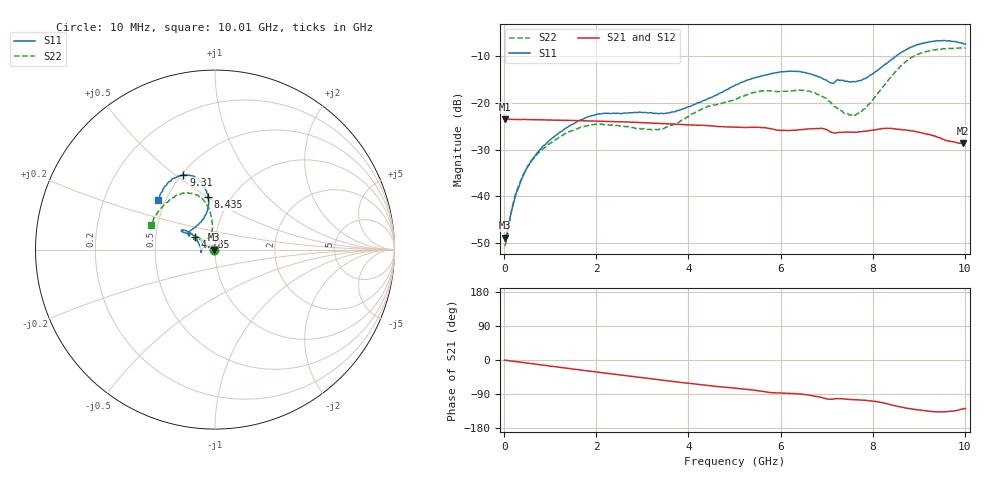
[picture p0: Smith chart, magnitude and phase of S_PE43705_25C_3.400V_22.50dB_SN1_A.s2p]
! Device ID: PE43705
! Serial: 1
! Insertion: A
! Impedance: 50 ohm
! Temp: 25C
! VDD: 3.400V
! Attenuation Step: 22.50dB
#  Hz  S  RI  R  50
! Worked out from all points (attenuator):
!   401 points, 10 MHz to 10.01 GHz, reference 50 ohm
!   highest |S21| = -23.53 dB at 10 MHz (marker M1); lowest = -28.7 dB at 9.96 GHz (marker M2)
!   lowest |S11| = -48.8 dB at 10 MHz (marker M3), VSWR 1.01, Z = 49.6 + j0.0396 ohm
!   |S11| at or under -10 dB: start of sweep to 8.518 GHz
!   |S22| runs from -50.6 to -8.3 dB; largest |S21 - S12| = 0.00078
!   S11 on the Smith chart (normalised r, x): 10 MHz: 0.99, +0.00; 4.785 GHz: 0.79, +0.12; 8.435 GHz: 0.79, +0.50; 9.31 GHz: 0.51, +0.53; 10.01 GHz: 0.45, +0.31
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1e7  -0.0036 0.000399  0.0666 -0.000213  0.0666 -0.000231  -0.00291 0.000506
6e7  -0.00344 0.00218  0.0664 -0.00125  0.0664 -0.00123  -0.00248 0.00251
2.6e8  -0.00513 0.00943  0.066 -0.00508  0.066 -0.00502  -0.00371 0.0104
5.35e8  -0.0124 0.0178  0.0652 -0.0102  0.0652 -0.0101  -0.00968 0.0192
1.01e9  -0.0346 0.0214  0.0626 -0.0185  0.0627 -0.0184  -0.0279 0.0245
1.685e9  -0.0655 0.00833  0.0572 -0.0289  0.0573 -0.0289  -0.0523 0.0168
2.185e9  -0.0765 -0.00715  0.052 -0.0359  0.0521 -0.0359  -0.0579 0.00703
3.36e9  -0.0761 -0.00613  0.0366 -0.0477  0.0366 -0.0476  -0.0502 0.0129
3.86e9  -0.0831 0.0182  0.0296 -0.0504  0.0297 -0.0503  -0.0587 0.0278
4.785e9  -0.1131 0.0727  0.0172 -0.0525  0.0173 -0.0525  -0.0822 0.0584
5.01e9  -0.1269 0.0856  0.0148 -0.0528  0.0148 -0.0528  -0.0888 0.0635
5.985e9  -0.1822 0.1091  0.00275 -0.0505  0.00293 -0.0505  -0.1099 0.0717
6.685e9  -0.1746 0.0955  -0.00394 -0.0527  -0.00384 -0.0527  -0.1145 0.0589
7.11e9  -0.1404 0.0801  -0.0113 -0.047  -0.0111 -0.047  -0.0815 0.0538
7.61e9  -0.0973 0.1359  -0.0125 -0.0468  -0.0122 -0.0468  -0.0368 0.0634
7.885e9  -0.0607 0.1764  -0.0148 -0.0477  -0.0144 -0.0479  -0.0215 0.0907
8.36e9  -0.0352 0.2749  -0.0243 -0.0474  -0.0241 -0.0473  -0.0196 0.1788
8.435e9  -0.0376 0.2923  -0.0257 -0.0462  -0.0258 -0.0462  -0.0237 0.1966
8.86e9  -0.0889 0.3858  -0.0316 -0.0387  -0.0314 -0.039  -0.0863 0.2935
9.31e9  -0.1761 0.4157  -0.032 -0.0307  -0.0318 -0.0309  -0.1876 0.3117
9.96e9  -0.3082 0.2948  -0.0233 -0.0284  -0.0239 -0.0285  -0.3467 0.1574
1.001e10  -0.316 0.278  -0.0233 -0.0295  -0.0229 -0.0294  -0.3585 0.1366
